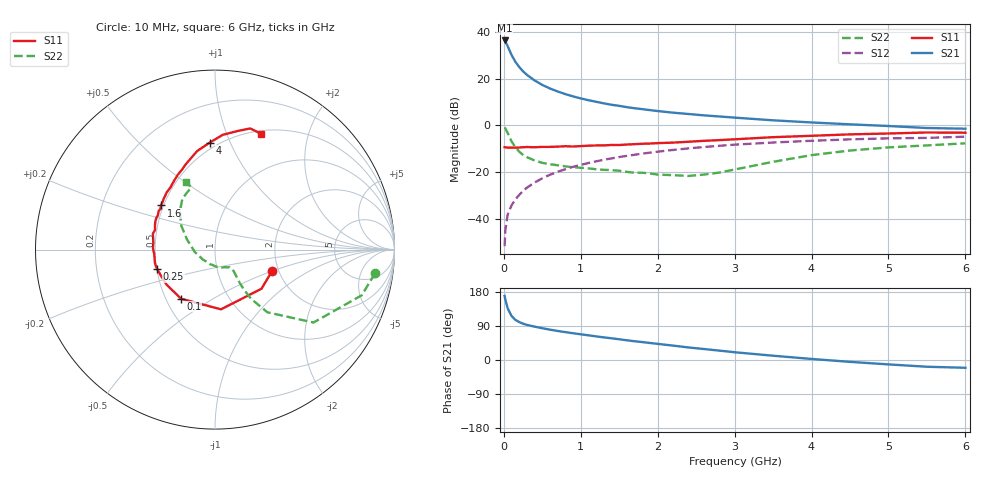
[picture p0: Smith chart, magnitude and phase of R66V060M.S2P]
! SIEMENS Small Signal Semiconductors
! BFR193
! Si NPN RF Bipolar Junction Transistor in SOT23
! VCE = 6 V  IC = 60 mA
! Common Emitter S-Parameters:  May  1996
# GHz  S  MA  R  50
!  f  S11  S21  S12  S22
! GHz  MAG  ANG  MAG  ANG  MAG  ANG  MAG  ANG
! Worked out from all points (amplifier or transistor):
!   36 points, 10 MHz to 6 GHz, reference 50 ohm
!   highest |S21| = 36.3 dB at 10 MHz (marker M1)
!   |S21| within 3 dB of that: start of sweep to 57.46 MHz
!   unconditionally stable (mu >= 1): 388.8 MHz to 2.092 GHz
!   at 250 MHz: K = 0.95, MSG = 25.6 dB, |S12| = -28.1 dB
!   at 1.4 GHz: K = 1.02, MAG = 10.6 dB, |S12| = -14.2 dB
!   at 6 GHz: K = 0.95, MSG = 1.7 dB, |S12| = -4.9 dB
!   S11 on the Smith chart (normalised r, x): 10 MHz: 1.85, -0.50; 100 MHz: 0.60, -0.37; 250 MHz: 0.50, -0.12; 1.6 GHz: 0.48, +0.28; 4 GHz: 0.45, +0.84; 6 GHz: 0.53, +1.33
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0.01  0.3399 -20.6  65.39 169.0  0.0026 78.5  0.9017 -8.4
0.02  0.3387 -40.1  62.21 159.0  0.0058 77.8  0.8562 -17.3
0.05  0.3344 -84.3  49.36 136.2  0.0124 70.2  0.683 -36.5
0.1  0.3327 -124.7  32.1 116.3  0.0193 68.1  0.4554 -50.1
0.15  0.333 -144.0  22.88 105.9  0.0261 69.8  0.3386 -53.8
0.2  0.3347 -154.5  17.65 100.1  0.0325 72.1  0.2744 -54.1
0.25  0.3401 -161.7  14.27 95.8  0.0393 73.0  0.2329 -53.5
0.3  0.3432 -166.8  12.01 92.7  0.0464 73.8  0.2087 -52.4
0.4  0.3397 -175.9  9.124 88.0  0.06 74.1  0.1771 -50.4
0.5  0.3458 178.6  7.314 83.8  0.0735 74.3  0.1575 -49.0
0.6  0.3456 173.7  6.135 80.1  0.0877 73.5  0.1472 -48.8
0.7  0.3501 169.8  5.298 76.6  0.1015 72.8  0.1398 -49.5
0.9  0.3518 161.8  4.155 70.6  0.1294 70.4  0.1268 -50.9
1.1  0.3669 155.2  3.447 65.1  0.1564 67.9  0.1201 -56.1
1.3  0.3717 148.8  2.951 59.7  0.1834 65.0  0.1117 -61.1
1.6  0.3882 140.7  2.446 52.0  0.2224 60.7  0.101 -73.3
2.2  0.4267 125.5  1.865 38.0  0.2975 51.7  0.086 -108.2
3.5  0.558 100.3  1.28 11.3  0.4289 31.3  0.1658 160.1
4  0.5971 92.8  1.152 2.8  0.4669 24.3  0.2305 144.6
4.5  0.6406 86.2  1.051 -4.9  0.5013 17.3  0.2891 132.6
5.5  0.7032 73.8  0.876 -17.8  0.5386 3.7  0.372 110.9
6  0.6944 68.4  0.847 -20.5  0.5716 -0.2  0.4123 113.2
